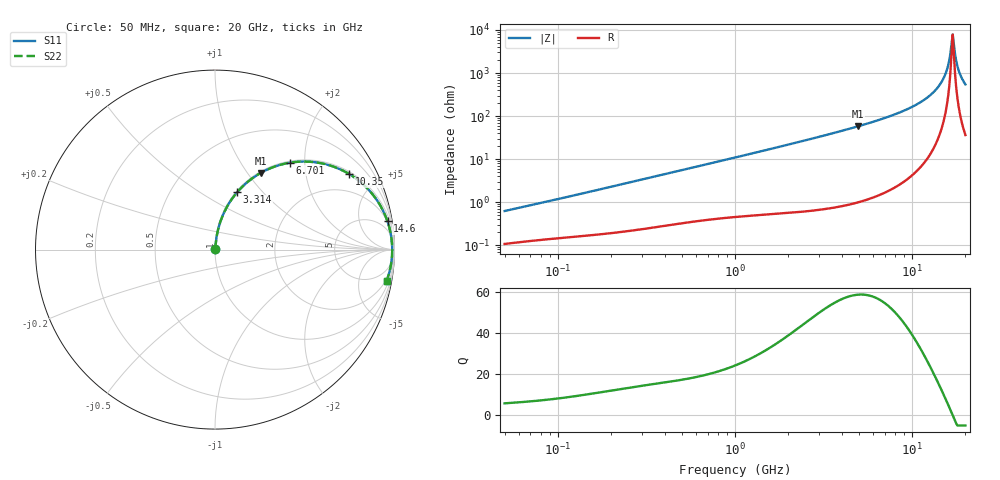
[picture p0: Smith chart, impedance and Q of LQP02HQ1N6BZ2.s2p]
!Murata Part Number: LQP02HQ1N6BZ2
!These Parameters are Measured in Series Mode Connection
!  o--[Z]--o
!Port1  Port2
!  o-------o
!Freq. Start=50[MHz] Stop=20[GHz], 401[Steps]
# Hz S RI R 50
!Freq.(Hz) S11(Real) S11(Imag) S21(Real) S21(Imag) S12(Real) S12(Imag) S22(Real) S22(Imag)
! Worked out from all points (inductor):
!   401 points, 50 MHz to 20 GHz, reference 50 ohm
!   read as one part in series: L = 1.91 nH near 51.52 MHz
!   highest Q = 58.5 at 4.967 GHz (marker M1), where L = 1.85 nH
!   self-resonance near 16.71 GHz
!   S11 on the Smith chart (normalised r, x): 50 MHz: 1.00, +0.01; 3.314 GHz: 1.01, +0.73; 6.701 GHz: 1.03, +1.69; 10.35 GHz: 1.09, +3.51; 14.6 GHz: 2, +12; 20 GHz: 2, -11
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5e7  0.0011 0.00611  0.9989 -0.00611  0.9989 -0.00611  0.0011 0.00611
1.364002e8  0.00186 0.0156  0.9981 -0.0156  0.9981 -0.0156  0.00186 0.0156
3.721004e8  0.00438 0.0412  0.9956 -0.0412  0.9956 -0.0412  0.00438 0.0412
1e9  0.016 0.1062  0.984 -0.1062  0.984 -0.1062  0.016 0.1062
2.728004e9  0.0868 0.2712  0.9132 -0.2712  0.9132 -0.2712  0.0868 0.2712
3.314454e9  0.1237 0.3198  0.8763 -0.3198  0.8763 -0.3198  0.1237 0.3198
4.966507e9  0.2546 0.4272  0.7454 -0.4272  0.7454 -0.4272  0.2546 0.4272
6.701223e9  0.4185 0.4844  0.5815 -0.4844  0.5815 -0.4844  0.4185 0.4844
7.442007e9  0.4909 0.4905  0.5091 -0.4905  0.5091 -0.4905  0.4909 0.4905
1.034674e10  0.7491 0.4202  0.2509 -0.4202  0.2509 -0.4202  0.7491 0.4202
1.276073e10  0.8974 0.2824  0.1026 -0.2824  0.1026 -0.2824  0.8974 0.2824
1.460232e10  0.9611 0.1575  0.0389 -0.1575  0.0389 -0.1575  0.9611 0.1575
1.573793e10  0.9807 0.0799  0.0193 -0.0799  0.0193 -0.0799  0.9807 0.0799
1.597544e10  0.9831 0.064  0.0169 -0.064  0.0169 -0.064  0.9831 0.064
1.646126e10  0.9863 0.0319  0.0137 -0.0319  0.0137 -0.0319  0.9863 0.0319
1.670968e10  0.9871 0.0157  0.0129 -0.0157  0.0129 -0.0157  0.9871 0.0157
1.696185e10  0.9874 -0.000456  0.0126 0.000456  0.0126 0.000456  0.9874 -0.000456
1.721783e10  0.9872 -0.0166  0.0128 0.0166  0.0128 0.0166  0.9872 -0.0166
1.800918e10  0.9833 -0.065  0.0167 0.065  0.0167 0.065  0.9833 -0.065
1.855685e10  0.9781 -0.0968  0.0219 0.0968  0.0219 0.0968  0.9781 -0.0968
1.940974e10  0.9665 -0.1435  0.0335 0.1435  0.0335 0.1435  0.9665 -0.1435
2e10  0.9563 -0.1737  0.0437 0.1737  0.0437 0.1737  0.9563 -0.1737
